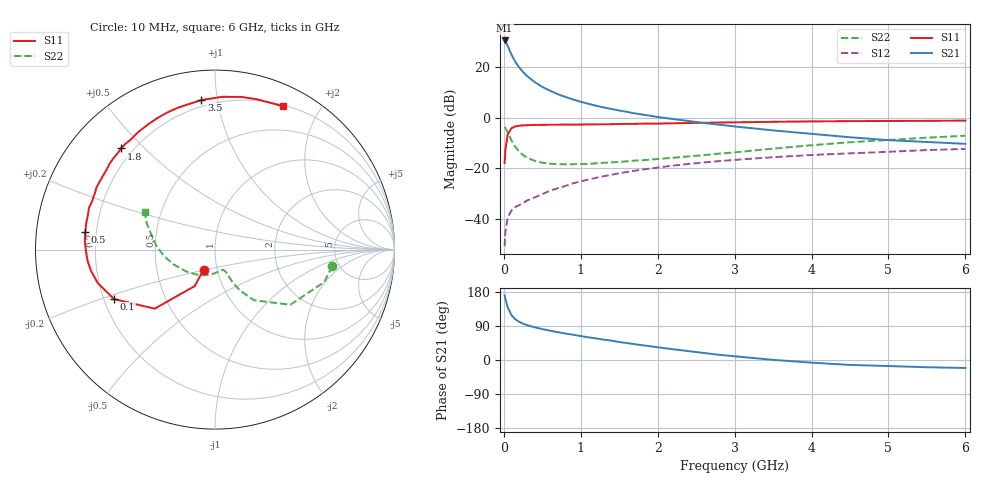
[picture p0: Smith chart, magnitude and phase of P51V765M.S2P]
! SIEMENS Small Signal Semiconductors
! BFP183
! Si NPN RF Bipolar Junction Transistor in SOT143
! VCE = 1.75 V  IC = 65 mA
! Common Emitter S-Parameters:  March  1996
# GHz  S  MA  R  50
!  f  S11  S21  S12  S22
! GHz  MAG  ANG  MAG  ANG  MAG  ANG  MAG  ANG
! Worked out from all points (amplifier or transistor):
!   36 points, 10 MHz to 6 GHz, reference 50 ohm
!   highest |S21| = 30.6 dB at 10 MHz (marker M1)
!   |S21| within 3 dB of that: start of sweep to 62.73 MHz
!   unconditionally stable (mu >= 1): start of sweep to 41.67 MHz; 127.6 MHz to end of sweep
!   at 250 MHz: K = 1.38, MAG = 22.2 dB, |S12| = -33.7 dB
!   at 1.4 GHz: K = 1.91, MAG = 7.5 dB, |S12| = -22.5 dB
!   at 6 GHz: K = 1.49, MAG = -3.1 dB, |S12| = -12.3 dB
!   S11 on the Smith chart (normalised r, x): 10 MHz: 0.86, -0.20; 100 MHz: 0.24, -0.22; 500 MHz: 0.16, +0.07; 1.8 GHz: 0.15, +0.43; 3.5 GHz: 0.16, +0.90; 6 GHz: 0.21, +1.56
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0.01  0.1294 -119.6  34.05 170.5  0.0029 57.3  0.6593 -8.0
0.02  0.2328 -119.1  32.9 161.4  0.0055 63.8  0.6355 -16.5
0.05  0.4704 -135.6  26.77 138.8  0.0107 56.4  0.5202 -36.2
0.1  0.6263 -153.9  17.74 118.2  0.0148 44.9  0.3551 -52.5
0.15  0.6792 -164.0  12.85 107.2  0.0174 43.8  0.2658 -58.6
0.2  0.7001 -170.1  9.932 100.7  0.0188 45.3  0.2148 -61.4
0.25  0.7121 -174.6  8.075 95.8  0.0207 48.1  0.1846 -62.4
0.3  0.7168 -178.0  6.777 92.2  0.0231 50.7  0.1637 -62.8
0.4  0.7261 176.8  5.132 86.3  0.0267 55.4  0.1416 -63.9
0.5  0.7296 172.3  4.104 81.6  0.0311 56.6  0.1298 -65.4
0.6  0.7324 168.3  3.457 77.4  0.0362 58.8  0.1242 -67.2
0.7  0.7336 164.8  2.952 73.5  0.0406 60.8  0.1213 -69.0
0.9  0.7359 158.6  2.315 66.6  0.0508 61.3  0.1214 -74.9
1.1  0.7453 152.3  1.9 59.7  0.0603 61.6  0.1233 -81.3
1.5  0.7572 141.0  1.399 47.4  0.0803 59.1  0.1346 -94.2
1.8  0.769 132.9  1.165 38.9  0.0949 56.5  0.1458 -105.4
2.2  0.7829 122.8  0.949 28.3  0.1137 52.4  0.1626 -119.6
2.8  0.8094 108.9  0.735 13.6  0.1398 45.4  0.1963 -140.1
3.5  0.8368 95.2  0.566 0.4  0.1668 37.6  0.2468 -160.9
4.5  0.8633 80.1  0.414 -13.0  0.1991 26.4  0.33 175.6
5.5  0.8744 69.2  0.334 -19.1  0.2309 16.6  0.4066 159.1
6  0.8834 64.6  0.307 -21.1  0.243 11.2  0.4431 152.0
